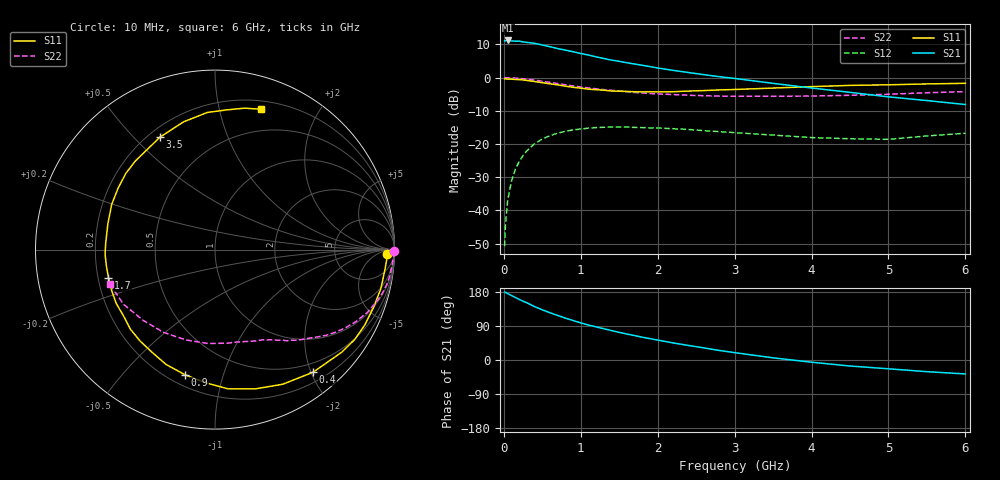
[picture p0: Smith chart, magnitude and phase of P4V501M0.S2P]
! SIEMENS Small Signal Semiconductors
! BFP182
! Si NPN RF Bipolar Junction Transistor in SOT143
! VCE = 0.5 V  IC = 1 mA
! Common Emitter S-Parameters:  March  1996
# GHz  S  MA  R  50
!  f  S11  S21  S12  S22
! GHz  MAG  ANG  MAG  ANG  MAG  ANG  MAG  ANG
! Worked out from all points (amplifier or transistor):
!   36 points, 10 MHz to 6 GHz, reference 50 ohm
!   highest |S21| = 11.2 dB at 50 MHz (marker M1)
!   |S21| within 3 dB of that: start of sweep to 818 MHz
!   unconditionally stable (mu >= 1): 2.426 GHz to end of sweep
!   at 250 MHz: K = 0.11, MSG = 17.1 dB, |S12| = -23.5 dB
!   at 1.4 GHz: K = 0.60, MSG = 10.1 dB, |S12| = -14.9 dB
!   at 6 GHz: K = 1.47, MAG = 0.3 dB, |S12| = -16.7 dB
!   S11 on the Smith chart (normalised r, x): 10 MHz: 36, -19; 400 MHz: 0.35, -2.03; 900 MHz: 0.26, -0.75; 1.7 GHz: 0.24, -0.12; 3.5 GHz: 0.24, +0.60; 6 GHz: 0.28, +1.34
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0.01  0.9578 -1.3  3.589 179.4  0.0029 86.3  0.997 -0.6
0.02  0.9604 -2.4  3.588 178.7  0.0058 88.4  0.9948 -1.2
0.05  0.9535 -6.6  3.635 175.1  0.0143 86.3  0.9946 -2.9
0.1  0.9496 -13.1  3.583 170.1  0.0279 81.2  0.9886 -5.9
0.15  0.9405 -19.8  3.544 165.0  0.0418 77.3  0.9839 -9.0
0.2  0.9344 -26.7  3.552 159.8  0.0547 73.1  0.9757 -11.8
0.4  0.8751 -51.3  3.29 140.8  0.1011 57.8  0.9187 -22.3
0.5  0.8396 -63.3  3.104 132.3  0.1192 50.7  0.8825 -27.0
0.6  0.8075 -74.0  2.926 124.7  0.1341 44.7  0.8477 -30.9
0.7  0.7799 -84.5  2.741 117.5  0.146 38.9  0.8143 -34.4
0.9  0.7167 -103.6  2.46 104.1  0.1634 29.2  0.7504 -40.4
1.1  0.6712 -121.4  2.192 92.3  0.1737 21.0  0.7004 -45.5
1.4  0.6295 -144.0  1.84 77.6  0.1807 10.6  0.6455 -51.9
1.7  0.6138 -165.2  1.605 64.5  0.1783 3.2  0.5985 -57.2
1.9  0.6129 -177.4  1.468 56.4  0.1756 -1.0  0.5774 -60.8
2.2  0.6139 166.5  1.289 45.1  0.1705 -6.1  0.5573 -66.0
2.8  0.6537 139.4  1.035 25.2  0.1541 -13.0  0.5277 -77.9
3.5  0.6975 116.1  0.821 5.7  0.1366 -16.0  0.5245 -94.3
4.5  0.7653 93.2  0.601 -15.9  0.1203 -11.0  0.5433 -122.0
5  0.7809 85.3  0.514 -23.2  0.1177 -4.2  0.5619 -135.5
5.5  0.805 78.2  0.452 -30.8  0.1326 -0.9  0.5934 -149.0
6  0.8224 72.0  0.394 -36.8  0.1457 -0.4  0.6172 -161.8
